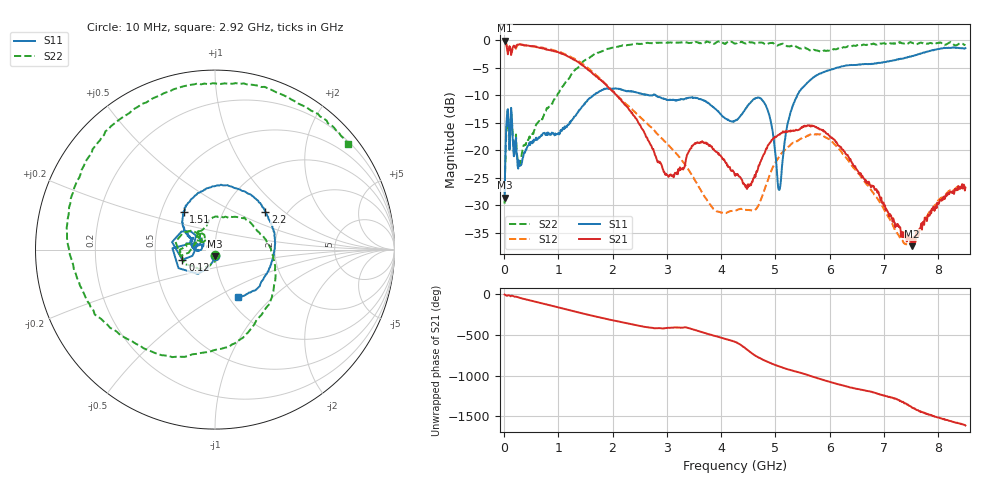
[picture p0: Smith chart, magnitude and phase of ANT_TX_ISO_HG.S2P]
!Agilent Technologies,E5071C,MY46523237,B.13.01
!Date: Tue Sep 12 16:55:46 2023
!Data & Calibration Information:
!Freq	S11:SOLT2(ON)	S21:SOLT2(ON)	S12:SOLT2(ON)	S22:SOLT2(ON)
!PortZ  Port1:50+j0  Port2:50+j0
!Above PortZ is port z conversion or system Z0 setting when saving the data.
!When reading, reference impedance value at option line is always used.
# Hz S dB R 50
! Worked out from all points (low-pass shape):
!   850 points, 10 MHz to 8.5 GHz, reference 50 ohm
!   highest |S21| = -0.07 dB at 10 MHz (marker M1); lowest = -37.4 dB at 7.52 GHz (marker M2)
!   |S21| within 3 dB of the highest: start of sweep to 1.202 GHz
!   lowest |S11| = -28.6 dB at 10 MHz (marker M3), VSWR 1.08, Z = 49.8 - j3.7 ohm
!   |S11| at or under -10 dB: start of sweep to 1.647 GHz; 2.66 GHz to 2.737 GHz (77.87 MHz wide, 2.89 % of centre); 2.794 GHz to 5.403 GHz (2.609 GHz wide, 63.7 % of centre)
!   |S22| runs from -29.7 to -0.2 dB; largest |S21 - S12| = 0.093
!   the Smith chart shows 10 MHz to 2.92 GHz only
!   S11 on the Smith chart (normalised r, x): 10 MHz: 1.00, -0.07; 120 MHz: 0.69, -0.08; 1.51 GHz: 0.65, +0.30; 2.2 GHz: 1.56, +0.75; 2.92 GHz: 1.10, -0.64
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1e7  -28.60 -91.1  -0.07 -3.3  -0.05 -3.5  -29.67 -87.7
1.2e8  -14.39 -162.7  -1.72 -24.7  -1.65 -24.8  -14.20 -169.8
6.3e8  -17.74 171.5  -1.32 -100.5  -1.22 -99.3  -14.86 92.3
1.03e9  -16.96 155.1  -2.31 -166.1  -2.15 -164.9  -9.13 -16.1
1.43e9  -12.17 137.3  -4.47 127.8  -4.19 128.8  -4.14 -105.8
1.51e9  -11.22 129.5  -5.07 114.6  -4.81 115.7  -3.52 -120.4
2.2e9  -9.10 36.8  -11.43 12.1  -11.13 17.8  -0.92 130.3
2.84e9  -10.28 -52.9  -22.02 -55.4  -17.18 -58.6  -0.50 48.3
2.92e9  -10.60 -64.3  -23.31 -60.4  -17.98 -67.6  -0.47 38.6
3.53e9  -10.51 -155.5  -18.79 -81.5  -25.64 -130.0  -0.36 -35.0
4.26e9  -14.61 23.8  -24.61 134.3  -30.91 -136.9  -0.62 -116.9
4.94e9  -16.03 159.3  -18.06 -134.2  -23.31 -151.3  -0.48 164.7
5.07e9  -27.19 47.8  -17.11 -165.4  -21.12 -173.8  -0.83 146.1
5.38e9  -10.50 -87.6  -16.25 130.0  -18.42 131.7  -1.17 98.8
5.67e9  -7.00 -130.0  -15.47 71.9  -17.02 77.4  -1.94 29.3
5.86e9  -5.90 -152.8  -16.27 32.1  -17.23 38.6  -2.05 -28.0
6.1e9  -5.12 -177.6  -18.22 -13.7  -19.03 -10.8  -1.66 -98.5
6.5e9  -4.47 143.8  -23.45 -81.9  -23.84 -78.1  -0.94 178.2
7.09e9  -3.82 89.2  -31.85 -178.6  -32.19 -177.0  -0.49 103.7
7.52e9  -2.88 44.9  -37.39 46.2  -36.36 49.7  -0.50 61.5
8.03e9  -1.56 -22.2  -28.95 -79.6  -28.77 -78.8  -0.44 11.6
8.5e9  -1.45 -103.1  -26.77 -170.7  -26.48 -168.0  -0.92 -36.7
